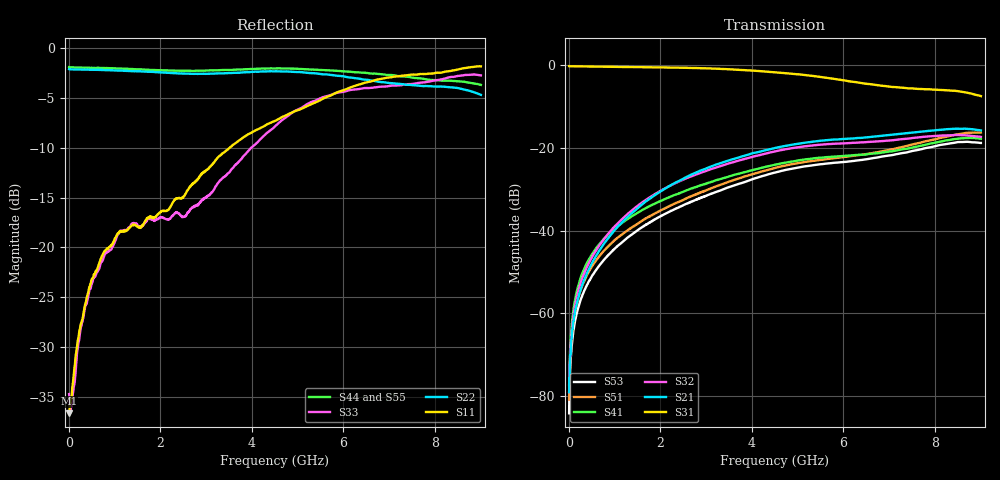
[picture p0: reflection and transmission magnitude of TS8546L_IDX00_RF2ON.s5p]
# GHz S DB R 50
! CMT, SN0916, 25263762, 26.7.0
! Date: 16.07.2026 08:28:49
! Data: Format
! Freq S1.1:dB/Ang S1.2:dB/Ang S1.3:dB/Ang S1.4:dB/Ang S1.5:dB/Ang
!  S2.1:dB/Ang S2.2:dB/Ang S2.3:dB/Ang S2.4:dB/Ang S2.5:dB/Ang
!  S3.1:dB/Ang S3.2:dB/Ang S3.3:dB/Ang S3.4:dB/Ang S3.5:dB/Ang
!  S4.1:dB/Ang S4.2:dB/Ang S4.3:dB/Ang S4.4:dB/Ang S4.5:dB/Ang
!  S5.1:dB/Ang S5.2:dB/Ang S5.3:dB/Ang S5.4:dB/Ang S5.5:dB/Ang
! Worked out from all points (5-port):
!   2001 points, 10 MHz to 9 GHz, reference 50 ohm
!   strongest paths, dB at 10 MHz, 2.257 GHz, 4.505 GHz, 6.753 GHz, 9 GHz:
!     S31: -0.2, -0.5, -1.6, -4.8, -7.4
!     S21: -79.1, -28.8, -20.0, -17.1, -15.7
!     S32: -79.1, -28.9, -20.8, -18.4, -17.3
!     S41: -77.5, -31.6, -24.0, -21.3, -17.8
!     S51: -80.9, -33.8, -24.8, -21.0, -16.3
!     S53: -84.3, -35.1, -26.0, -22.3, -18.8
!   lowest |S11| = -36.7 dB at 10 MHz (marker M1), VSWR 1.03, Z = 51.5 - j0.0221 ohm
!   |S11| at or under -10 dB: start of sweep to 3.516 GHz
